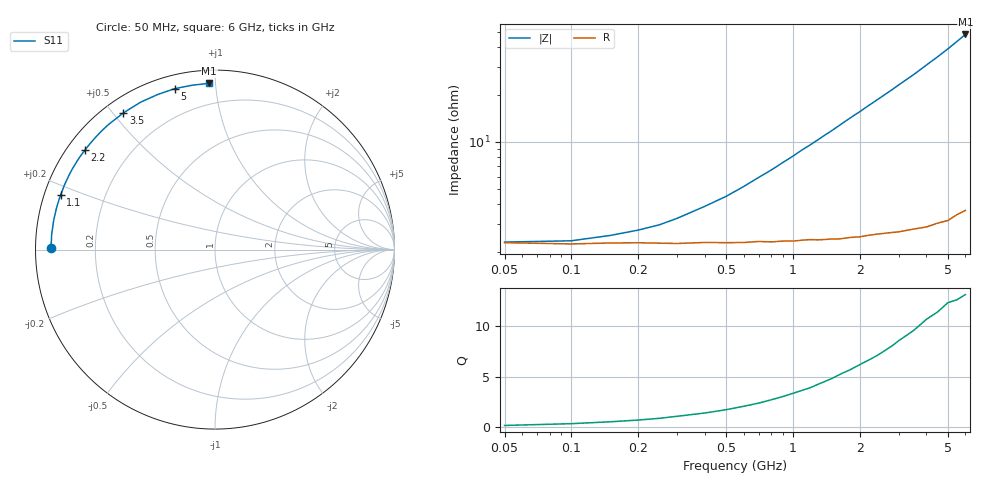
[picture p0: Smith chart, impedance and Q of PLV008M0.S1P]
! Infineon Technologies  Discrete & RF Semiconductors
! BAR 64-04W /-05W /-06W
! Si PIN Diode in SOT323
! IF = 8 mA
! S-Parameters:  October  2008
# GHz  S  MA  R  50
!  f  S11
! GHz  MAG  ANG
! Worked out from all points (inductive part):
!   34 points, 50 MHz to 6 GHz, reference 50 ohm
!   read as one part to ground: L = 1.23 nH near 900 MHz
!   highest Q = 13.1 at 6 GHz (marker M1), where L = 1.28 nH
!   S11 on the Smith chart (normalised r, x): 50 MHz: 0.05, +0.01; 1.1 GHz: 0.05, +0.17; 2.2 GHz: 0.05, +0.34; 3.5 GHz: 0.06, +0.53; 5 GHz: 0.06, +0.78; 6 GHz: 0.07, +0.96
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0.05  0.9127 179.3
0.1  0.9143 178.4
0.15  0.9132 177.4
0.25  0.9134 175.6
0.3  0.9139 174.6
0.6  0.9132 169.3
0.8  0.913 165.8
0.9  0.9124 164.0
1  0.9128 162.3
1.1  0.9121 160.5
1.2  0.9118 158.9
1.3  0.9126 157.2
1.4  0.9126 155.5
1.6  0.9132 152.2
1.7  0.913 150.5
1.9  0.9128 147.3
2  0.9131 145.8
2.2  0.9126 142.6
2.4  0.9128 139.6
2.6  0.9135 136.6
2.8  0.9142 133.7
3  0.9153 130.7
3.5  0.9169 123.8
4  0.9199 116.8
4.5  0.9213 110.3
5  0.9244 104.0
5.5  0.9247 97.8
6  0.9269 92.0
